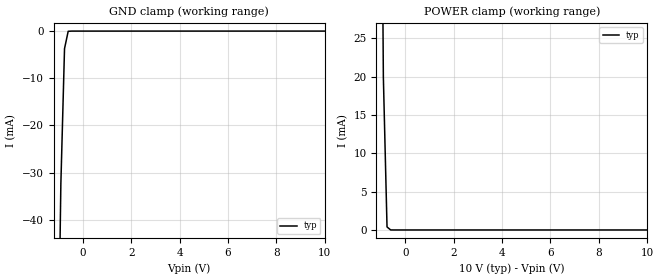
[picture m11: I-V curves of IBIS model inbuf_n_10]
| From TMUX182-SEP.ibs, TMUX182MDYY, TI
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| inbuf_n_10
[Model]   inbuf_n_10
Model_type   Input
Vinl = 0.8
Vinh = 1.35
|   typ   min   max
C_comp   6.362683e-13   NA   NA
[Voltage Range]   10   NA   NA
[Temperature Range]   27   NA   NA
[Power Clamp Reference]   10   NA   NA
[GND Clamp Reference]   0   NA   NA
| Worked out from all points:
|   GND clamp passes 1 mA (typ) near -0.65 V on its own axis
|   POWER clamp passes 1 mA (typ) near -0.76 V on its own axis
[GND Clamp]
|   Voltage   I(typ)   I(min)   I(max)
-5V       -2.674A    NA         NA
-1.061V   -87.09mA   NA         NA
-909.1mV  -32.43mA   NA         NA
-757.6mV  -3.722mA   NA         NA
-606.1mV  -41.8uA    NA         NA
10V       66.5nA     NA         NA
[POWER Clamp]
|   Voltage   I(typ)   I(min)   I(max)
-5V       3.29A      NA         NA
-1.061V   85.94mA    NA         NA
-909.1mV  19.94mA    NA         NA
-757.6mV  393.8uA    NA         NA
-606.1mV  1.601uA    NA         NA
10V       -416.4nA   NA         NA
